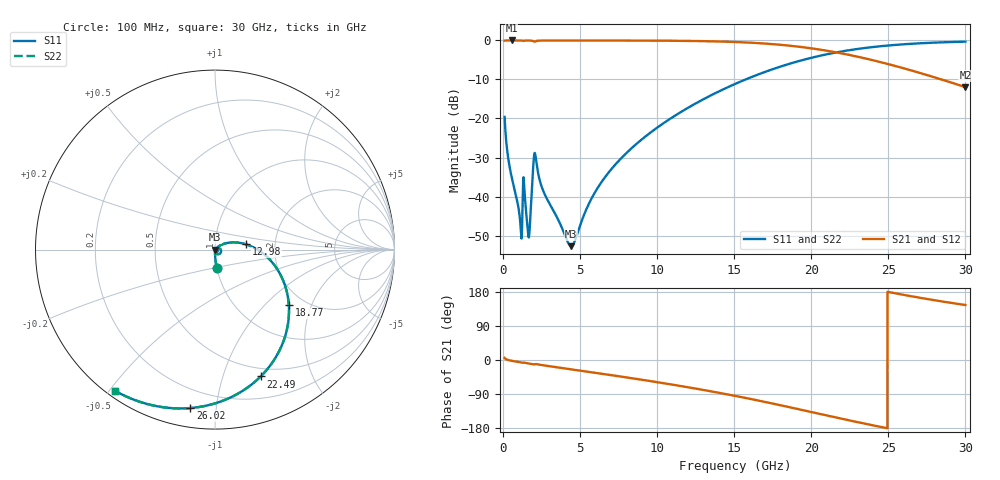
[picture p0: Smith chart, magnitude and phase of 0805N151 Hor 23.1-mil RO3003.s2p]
# GHz S MA R 50
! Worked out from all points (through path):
!   3201 points, 100 MHz to 30 GHz, reference 50 ohm
!   highest |S21| = -0.01 dB at 548.5 MHz (marker M1); lowest = -12.0 dB at 30 GHz (marker M2)
!   group delay of S21, straight-line fit = 20.9 ps
!   lowest |S11| = -52.7 dB at 4.417 GHz (marker M3), VSWR 1.00, Z = 50.2 - j0.101 ohm
!   |S11| at or under -10 dB: start of sweep to 15.74 GHz
!   |S22| runs from -52.7 to -0.3 dB; largest |S21 - S12| = 0
!   S11 on the Smith chart (normalised r, x): 100 MHz: 1.00, -0.21; 12.98 GHz: 1.42, +0.09; 18.77 GHz: 1.66, -1.40; 22.49 GHz: 0.41, -1.34; 26.02 GHz: 0.10, -0.85; 30 GHz: 0.02, -0.52
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0.1  0.1046 -84.4  0.9942 5.4  0.9942 5.4  0.1046 -84.4
0.5485  0.01806 -90.0  0.9992 -2.1  0.9992 -2.1  0.01806 -90.0
1.099781  0.005028 -80.3  0.9986 -5.9  0.9986 -5.9  0.005028 -80.3
1.398781  0.01094 -71.5  0.9951 -7.3  0.9951 -7.3  0.01094 -71.5
1.651063  0.003029 -32.2  0.9971 -9.2  0.9971 -9.2  0.003029 -32.2
1.763187  0.005162 23.2  0.9956 -10.1  0.9956 -10.1  0.005162 23.2
1.978094  0.02804 9.1  0.9737 -11.7  0.9737 -11.7  0.02804 9.1
2.108906  0.03264 -50.6  0.9747 -10.6  0.9747 -10.6  0.03264 -50.6
2.6415  0.01138 -87.4  0.9966 -14.2  0.9966 -14.2  0.01138 -87.4
4.416812  0.002314 -25.8  0.9975 -24.6  0.9975 -24.6  0.002314 -25.8
5.089563  0.004792 31.4  0.9974 -28.5  0.9974 -28.5  0.004792 31.4
5.865094  0.01048 42.9  0.9972 -33.1  0.9972 -33.1  0.01048 42.9
6.911594  0.02106 43.2  0.9968 -39.3  0.9968 -39.3  0.02106 43.2
10.06978  0.07813 28.4  0.993 -58.9  0.993 -58.9  0.07813 28.4
12.97569  0.1754 9.6  0.9795 -78.9  0.9795 -78.9  0.1754 9.6
15.05  0.2768 -5.7  0.9549 -94.6  0.9549 -94.6  0.2768 -5.7
18.76881  0.5149 -37.0  0.8494 -126.2  0.8494 -126.2  0.5149 -37.0
20.03956  0.6017 -48.4  0.7903 -137.6  0.7903 -137.6  0.6017 -48.4
22.48763  0.7511 -70.2  0.6508 -159.5  0.6508 -159.5  0.7511 -70.2
25.01978  0.8624 -91.2  0.4959 179.3  0.4959 179.3  0.8624 -91.2
26.01956  0.8935 -98.9  0.4384 171.7  0.4384 171.7  0.8935 -98.9
30  0.9643 -125.5  0.2523 145.1  0.2523 145.1  0.9643 -125.5
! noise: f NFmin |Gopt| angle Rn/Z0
0.1  0.0003985  0.8498  0.6426  0.0005651
3.417  0.006766  0.7211  19.13  0.004679
6.743  0.01025  0.6576  37.09  0.005161
10.06  0.01423  0.6454  53.97  0.00611
13.39  0.01876  0.6526  69.67  0.007073
16.7  0.02427  0.6727  84.18  0.00811
20.03  0.03143  0.7029  97.79  0.009322
23.35  0.04125  0.7416  110.7  0.01082
26.67  0.0557  0.7874  123.4  0.0127
30  0.07851  0.8369  136.1  0.01493
